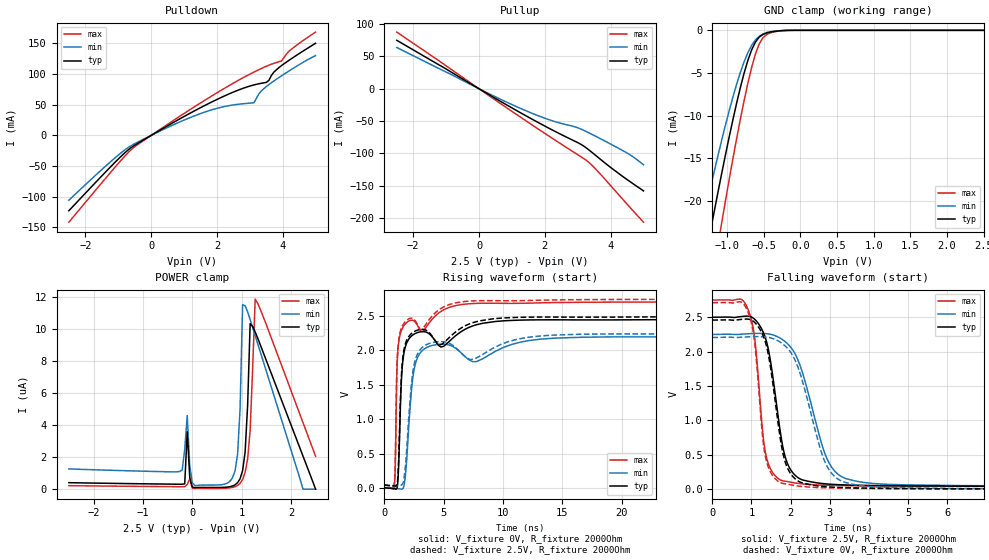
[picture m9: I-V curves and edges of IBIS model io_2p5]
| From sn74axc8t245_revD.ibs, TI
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|   io_2p5 Model
[Model]   io_2p5
Model_type   I/O
Polarity   Non-Inverting
Enable   Active-High
Vinl = 0.75
Vinh = 1.75
Vmeas = 1.25
Vref = 0
Cref = 2pF
Rref = 100000
|   typ   min   max
C_comp   1.540pF   1.379pF   1.785pF
| Where Nom  PVT is Nominal Process, 2.5V, 27C
|   Fast PVT is Strong Process,  2.75V, -40C
|   Slow PVT is Weak Process,   2.25, 125C
[Voltage Range]   2.5   2.25   2.75
|Junction Temperature
[Temperature Range]   27   125   -40
[Pullup Reference]   2.5   2.25   2.75
[Pulldown Reference]   0   0   0
[Power Clamp Reference]   2.5   2.25   2.75
[GND Clamp Reference]   0   0   0
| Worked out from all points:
|   slope of the pulldown table from 0 to 0.375 V, typ, clamps not added: 31.8 ohm
|   slope of the pullup table from 0 to 0.375 V, typ, clamps not added: 33.3 ohm
|   GND clamp passes 1 mA (typ) near -0.58 V on its own axis
|   falling waveform, V_fixture 2.5V, R_fixture 2000Ohm: 20-80 % time 394ps typ, 665ps min, 263ps max; typ from 2.5 V to 0.039 V
|   rising waveform, V_fixture 0V, R_fixture 2000Ohm: 20-80 % time 419ps typ, 664ps min, 310ps max; typ from 0 V to 2.46 V
|   rising waveform, V_fixture 2.5V, R_fixture 2000Ohm: 20-80 % time 423ps typ, 672ps min, 314ps max; typ from 0.039 V to 2.5 V
|   falling waveform, V_fixture 0V, R_fixture 2000Ohm: 20-80 % time 389ps typ, 653ps min, 261ps max; typ from 2.46 V to 0 V
[Pulldown]
|Voltage   I(typ)   I(min)   I(max)
-2.5V     -122.7mA   -105.6mA   -141.4mA
-1.132V   -45.74mA   -38.18mA   -54mA
-524mV    -16.87mA   -14.27mA   -19.51mA
1.604V    48.02mA    37.53mA    56.35mA
2.288V    65.71mA    47.72mA    78.59mA
3.124V    82.24mA    53.17mA    103.2mA
3.276V    84.17mA    67.77mA    107.2mA
3.504V    86.42mA    79.65mA    112.7mA
3.732V    103.1mA    88.7mA     117.5mA
3.96V     113.6mA    96.99mA    121.2mA
4.264V    125mA      107.5mA    140.4mA
5V        150.2mA    130.1mA    168.4mA
[GND Clamp]
|Voltage   I(typ)   I(min)   I(max)
-2.5V     -85.92mA   -72.48mA   -101.3mA
-1.378V   -30.54mA   -24.33mA   -38.61mA
-1.327V   -28.17mA   -22.33mA   -35.87mA
-1.225V   -23.5mA    -18.43mA   -30.45mA
-1.174V   -21.22mA   -16.53mA   -27.78mA
-1.072V   -16.75mA   -12.86mA   -22.53mA
-868mV    -8.5mA     -6.29mA    -12.65mA
-715mV    -3.502mA   -2.603mA   -6.167mA
-613mV    -1.378mA   -1.131mA   -2.784mA
-511mV    -483.8uA   -430.3uA   -873.9uA
-205mV    -15.33uA   -14.93uA   -16.6uA
2.5V      0A         0A         0A
[Pullup]
|Voltage   I(typ)   I(min)   I(max)
-2.5V     75.07mA    64.01mA    87.79mA
212mV     -6.383mA   -5.369mA   -7.473mA
1.2V      -35.41mA   -29.04mA   -41.88mA
2.036V    -58.73mA   -46.27mA   -70.32mA
2.948V    -82.13mA   -59.49mA   -100.4mA
3.252V    -91.33mA   -66.08mA   -110.6mA
3.632V    -106.8mA   -75.81mA   -129mA
4.468V    -139.5mA   -98.53mA   -176.9mA
4.696V    -147.6mA   -105.9mA   -189.8mA
5V        -158.2mA   -117.8mA   -206.7mA
[POWER Clamp]
|   Voltage   I(typ)   I(min)   I(max)
-2.5V     405.1nA    1.265uA    219.4nA
-254mV    308nA      1.102uA    153.5nA
-152mV    332.4nA    2.482uA    152.6nA
-101mV    3.587uA    4.599uA    287.5nA
1mV       136.9nA    414.1nA    63.89nA
766mV     156.4nA    497.3nA    83.48nA
919mV     401.6nA    2.172uA    232.7nA
1.021V    1.162uA    11.52uA    603.1nA
1.123V    5.246uA    11.07uA    1.901uA
1.174V    10.34uA    10.59uA    3.674uA
1.276V    9.816uA    9.587uA    11.87uA
2.5V      0A         0A         2.058uA
[Ramp]
R_load = 3000
|   typ   min   max
dV/dt_r   1.349/0.399n   1.191/0.672n   1.507/0.280n
dV/dt_f   1.357/0.421n   1.198/0.757n   1.511/0.271n
[Falling Waveform]
V_fixture = 2.5V
V_fixture_min = 2.25V
V_fixture_max = 2.75V
R_fixture = 2000Ohm
C_fixture = 0F
|   Time   V(typ)   V(min)   V(max)
0s        2.5V       2.25V      2.75V
895ps     2.516V     2.259V     2.637V
1.08ns    2.471V     2.264V     2.203V
1.248ns   2.342V     2.265V     1.077V
1.432ns   2.031V     2.257V     368.1mV
1.858ns   478mV      2.147V     116.7mV
2.331ns   130.3mV    1.643V     75.11mV
3.05ns    70.61mV    318mV      55.24mV
4.447ns   50.85mV    71.2mV     44.89mV
50ns      38.86mV    41.52mV    37.31mV
[Rising Waveform]
|Gnd
V_fixture = 0V
V_fixture_min = 0V
V_fixture_max = 0V
R_fixture = 2000Ohm
C_fixture = 0F
|   Time   V(typ)   V(min)   V(max)
0s        70.9nV     319.6nV    38nV
840ps     -13.14mV   -6.658mV   34.04mV
907ps     -16.63mV   -6.713mV   284.8mV
1.077ns   11.74mV    -9.559mV   1.827V
1.435ns   1.579V     -18.55mV   2.295V
1.768ns   2.056V     183.4mV    2.388V
2.321ns   2.216V     1.497V     2.44V
2.7ns     2.255V     1.857V     2.389V
5.722ns   2.173V     2.062V     2.641V
50ns      2.457V     2.204V     2.71V
[Rising Waveform]
V_fixture = 2.5V
V_fixture_min = 2.25V
V_fixture_max = 2.75V
R_fixture = 2000Ohm
C_fixture = 0F
|   Time   V(typ)   V(min)   V(max)
0s        38.71mV    41.33mV    37.21mV
841ps     28.11mV    35.96mV    79.52mV
1.076ns   66.17mV    35.82mV    1.868V
1.405ns   1.537V     39.22mV    2.314V
1.772ns   2.1V       317.3mV    2.421V
2.288ns   2.248V     1.535V     2.47V
2.646ns   2.287V     1.889V     2.419V
5.552ns   2.202V     2.098V     2.673V
10.45ns   2.477V     2.128V     2.723V
50ns      2.498V     2.247V     2.748V
[Falling Waveform]
V_fixture = 0V
V_fixture_min = 0V
V_fixture_max = 0V
R_fixture = 2000Ohm
C_fixture = 0F
|   Time   V(typ)   V(min)   V(max)
0s        2.459V     2.207V     2.712V
906ps     2.473V     2.215V     2.581V
1.085ns   2.423V     2.218V     2.116V
1.238ns   2.302V     2.217V     1.069V
1.408ns   2.022V     2.209V     358.4mV
1.828ns   464.2mV    2.099V     81.7mV
2.301ns   91.23mV    1.574V     38.71mV
2.999ns   31.9mV     268.3mV    18.58mV
4.035ns   14.77mV    37.57mV    9.354mV
50ns      152.1uV    197.7uV    100.1uV
